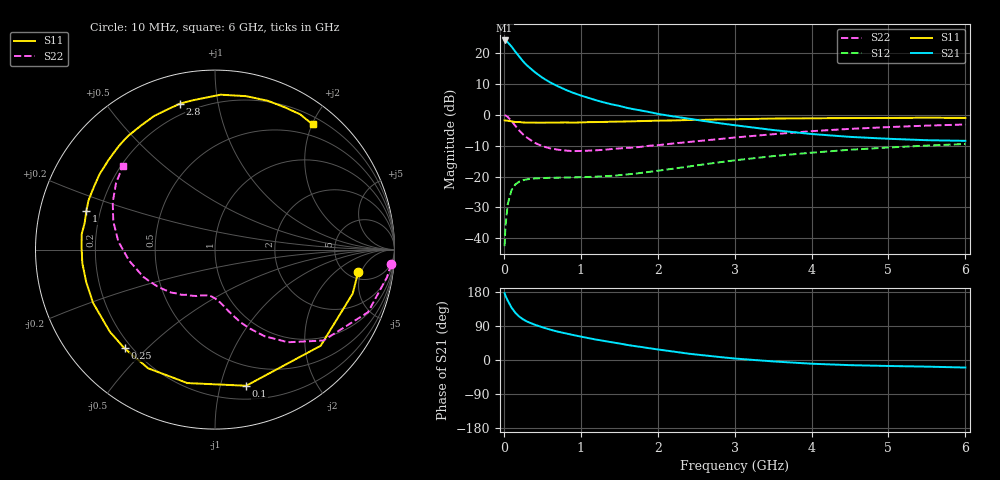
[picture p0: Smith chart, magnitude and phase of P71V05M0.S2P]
! SIEMENS Small Signal Semiconductors
! BFP196
! Si NPN RF Bipolar Junction Transistor in SOT143
! VCE = 1 V  IC = 5 mA
! Common Emitter S-Parameters:  May  1996
# GHz  S  MA  R  50
!  f  S11  S21  S12  S22
! GHz  MAG  ANG  MAG  ANG  MAG  ANG  MAG  ANG
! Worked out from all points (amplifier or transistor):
!   36 points, 10 MHz to 6 GHz, reference 50 ohm
!   highest |S21| = 24.0 dB at 10 MHz (marker M1)
!   |S21| within 3 dB of that: start of sweep to 131 MHz
!   unconditionally stable (mu >= 1): 1.103 GHz to end of sweep
!   at 250 MHz: K = 0.26, MSG = 19.2 dB, |S12| = -21.2 dB
!   at 1.4 GHz: K = 1.16, MAG = 9.1 dB, |S12| = -19.8 dB
!   at 6 GHz: K = 1.04, MAG = -0.7 dB, |S12| = -9.5 dB
!   S11 on the Smith chart (normalised r, x): 10 MHz: 6.11, -4.42; 100 MHz: 0.31, -1.21; 250 MHz: 0.17, -0.43; 1 GHz: 0.15, +0.14; 2.8 GHz: 0.14, +0.78; 6 GHz: 0.31, +2.01
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0.01  0.807 -9.0  15.77 176.3  0.0075 86.0  0.9845 -4.8
0.02  0.8053 -17.7  15.43 170.2  0.015 80.9  0.9706 -9.1
0.05  0.796 -42.3  14.73 156.9  0.0355 68.7  0.9209 -22.3
0.1  0.7782 -77.1  12.6 138.4  0.0605 52.6  0.7881 -40.0
0.15  0.7594 -101.7  10.37 124.4  0.0748 41.3  0.6569 -51.8
0.2  0.759 -119.4  8.673 114.7  0.0826 34.4  0.555 -60.3
0.25  0.7463 -132.5  7.25 107.3  0.087 29.3  0.4775 -66.5
0.3  0.7434 -142.0  6.254 101.7  0.0902 26.2  0.4266 -70.9
0.4  0.7415 -156.4  4.886 93.3  0.0932 22.1  0.3511 -77.6
0.5  0.7401 -166.0  3.953 86.4  0.0943 19.8  0.3085 -82.5
0.6  0.7431 -174.2  3.326 80.3  0.0954 18.8  0.2857 -86.3
0.7  0.7434 179.0  2.879 74.9  0.0956 18.6  0.2714 -90.1
0.8  0.7475 173.4  2.53 70.4  0.0966 18.7  0.263 -93.6
1  0.748 163.4  2.038 61.8  0.0976 20.2  0.2587 -99.9
1.1  0.7562 158.9  1.863 57.7  0.0984 21.4  0.2616 -103.1
1.6  0.7754 139.9  1.286 40.0  0.1081 28.2  0.2901 -118.1
2.2  0.8051 120.6  0.937 22.4  0.1337 34.3  0.3415 -135.4
2.8  0.8365 103.4  0.728 8.0  0.1696 34.4  0.4027 -153.5
3.5  0.8637 87.9  0.564 -3.7  0.2135 28.9  0.4822 -172.6
4.5  0.8797 70.5  0.437 -13.6  0.2708 17.9  0.5885 164.4
5.5  0.8906 57.8  0.386 -17.5  0.3161 5.9  0.6641 146.1
6  0.8844 52.1  0.377 -19.9  0.3354 -0.5  0.6926 138.0
